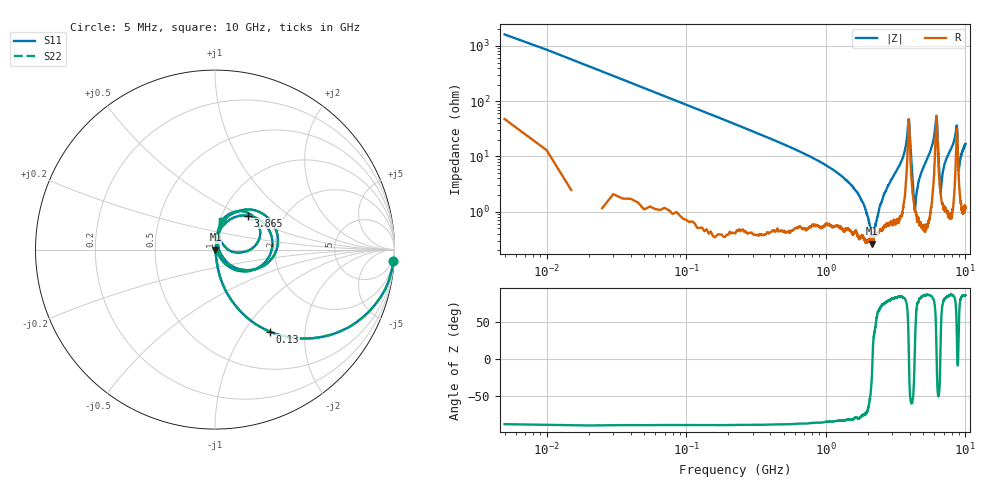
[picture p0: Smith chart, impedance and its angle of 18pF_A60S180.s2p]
! Amotech Co.,Ltd.
! http://www.amotech.co.kr/
! Part Number: A60S180
! These Parameters are Measured in Series Mode Connection
! Operation Temp=25[degC], DC Bias Voltage=0[V]
! Freq. Start=5[MHz] Stop=10[GHz], 2000[Steps]
! Date: Monday, July 13, 2020, 01:37:32
# GHZ S RI R 50.000000
!Freq.(Hz) S11(Real) S11(Imag) S21(Real) S21(Imag) S12(Real) S12(Imag) S22(Real) S22(Imag)
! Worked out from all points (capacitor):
!   2000 points, 5 MHz to 10 GHz, reference 50 ohm
!   read as one part in series: C = 18.4 pF near 55 MHz
!   lowest |Z| = 264 mohm at 2.155 GHz (marker M1)
!   series resonance near 2.162 GHz, so ESL is about 290 pH
!   S11 on the Smith chart (normalised r, x): 5 MHz: 2, -32; 130 MHz: 1.01, -1.33; 3.865 GHz: 1.32, +0.54; 10 GHz: 1.02, +0.34
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0.005  0.9944 -0.0616  0.00564 0.0616  0.00564 0.0616  0.9944 -0.0616
0.07  0.6021 -0.4847  0.3979 0.4847  0.3979 0.4847  0.6021 -0.4847
0.13  0.307 -0.4574  0.693 0.4574  0.693 0.4574  0.307 -0.4574
0.405  0.0452 -0.1976  0.9548 0.1976  0.9548 0.1976  0.0452 -0.1976
1.675  0.00464 -0.022  0.9954 0.022  0.9954 0.022  0.00464 -0.022
2.155  0.00261 -0.000336  0.9974 0.000336  0.9974 0.000336  0.00261 -0.000336
2.615  0.0057 0.0199  0.9943 -0.0199  0.9943 -0.0199  0.0057 0.0199
3.34  0.011 0.0645  0.989 -0.0645  0.989 -0.0645  0.011 0.0645
3.865  0.182 0.1894  0.818 -0.1894  0.818 -0.1894  0.182 0.1894
3.97  0.2422 -0.1003  0.7578 0.1003  0.7578 0.1003  0.2422 -0.1003
4.34  0.0103 0.00194  0.9897 -0.00194  0.9897 -0.00194  0.0103 0.00194
5.005  0.00878 0.0632  0.9912 -0.0632  0.9912 -0.0632  0.00878 0.0632
5.895  0.0622 0.1752  0.9378 -0.1752  0.9378 -0.1752  0.0622 0.1752
6.195  0.3479 0.08  0.6521 -0.08  0.6521 -0.08  0.3479 0.08
6.315  0.176 -0.1144  0.824 0.1144  0.824 0.1144  0.176 -0.1144
6.58  0.0254 -0.00888  0.9746 0.00888  0.9746 0.00888  0.0254 -0.00888
6.67  0.0195 0.0136  0.9805 -0.0136  0.9805 -0.0136  0.0195 0.0136
7.09  0.0164 0.0699  0.9836 -0.0699  0.9836 -0.0699  0.0164 0.0699
8.335  0.0567 0.1826  0.9433 -0.1826  0.9433 -0.1826  0.0567 0.1826
8.68  0.2505 0.1117  0.7495 -0.1117  0.7495 -0.1117  0.2505 0.1117
8.965  0.0407 0.0346  0.9593 -0.0346  0.9593 -0.0346  0.0407 0.0346
10  0.0389 0.161  0.9611 -0.161  0.9611 -0.161  0.0389 0.161
